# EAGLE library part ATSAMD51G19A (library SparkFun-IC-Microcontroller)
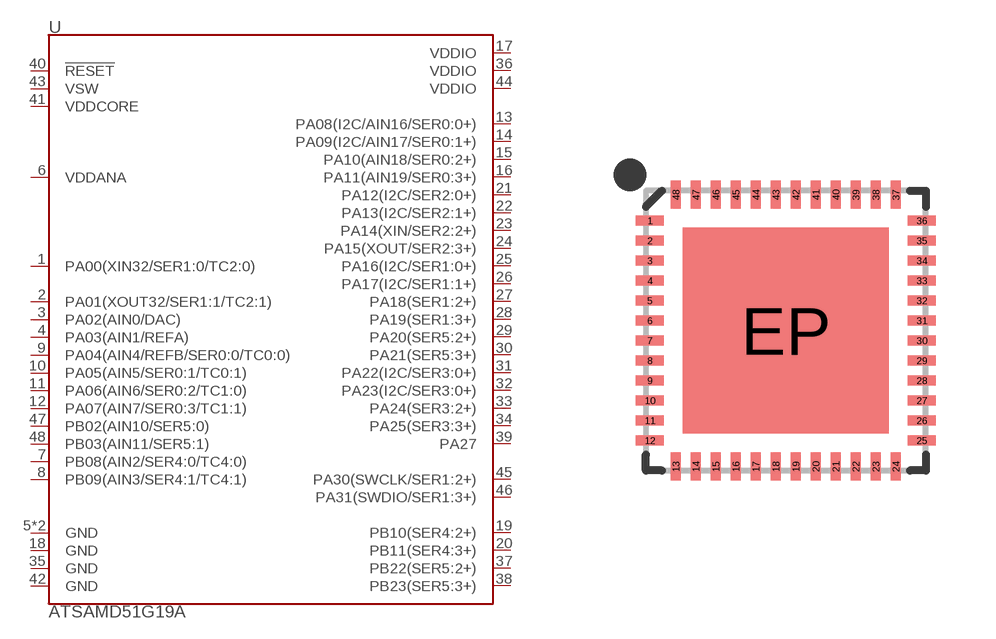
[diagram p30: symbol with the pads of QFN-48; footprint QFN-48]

Designator prefix -

## ATSAMD51G19A  [QFN-48]
1  PA00(XIN32/SER1:0/TC2:0)
2  PA01(XOUT32/SER1:1/TC2:1)
3  PA02(AIN0/DAC)
4  PA03(AIN1/REFA)
5  GND
6  VDDANA
7  PB08(AIN2/SER4:0/TC4:0)
8  PB09(AIN3/SER4:1/TC4:1)
9  PA04(AIN4/REFB/SER0:0/TC0:0)
10  PA05(AIN5/SER0:1/TC0:1)
11  PA06(AIN6/SER0:2/TC1:0)
12  PA07(AIN7/SER0:3/TC1:1)
13  PA08(I2C/AIN16/SER0:0+)
14  PA09(I2C/AIN17/SER0:1+)
15  PA10(AIN18/SER0:2+)
16  PA11(AIN19/SER0:3+)
17  VDDIO
18  GND
19  PB10(SER4:2+)
20  PB11(SER4:3+)
21  PA12(I2C/SER2:0+)
22  PA13(I2C/SER2:1+)
23  PA14(XIN/SER2:2+)
24  PA15(XOUT/SER2:3+)
25  PA16(I2C/SER1:0+)
26  PA17(I2C/SER1:1+)
27  PA18(SER1:2+)
28  PA19(SER1:3+)
29  PA20(SER5:2+)
30  PA21(SER5:3+)
31  PA22(I2C/SER3:0+)
32  PA23(I2C/SER3:0+)
33  PA24(SER3:2+)
34  PA25(SER3:3+)
35  GND
36  VDDIO
37  PB22(SER5:2+)
38  PB23(SER5:3+)
39  PA27
40  !RESET!
41  VDDCORE
42  GND
43  VSW
44  VDDIO
45  PA30(SWCLK/SER1:2+)
46  PA31(SWDIO/SER1:3+)
47  PB02(AIN10/SER5:0)
48  PB03(AIN11/SER5:1)
EP  GND

## Footprint QFN-48 (pad centres in mm)
48-pin QFN (7x7mm, 0.5mm pitch) Used on: ATSAMD21G
smd 0.7 x 0.25: 1 -3.4,2.75; 2 -3.4,2.25; 3 -3.4,1.75; 4 -3.4,1.25; 5 -3.4,0.75; 6 -3.4,0.25; 7 -3.4,-0.25; 8 -3.4,-0.75; 9 -3.4,-1.25; 10 -3.4,-1.75; 11 -3.4,-2.25; 12 -3.4,-2.75; 25 3.4,-2.75; 26 3.4,-2.25; 27 3.4,-1.75; 28 3.4,-1.25; 29 3.4,-0.75; 30 3.4,-0.25; 31 3.4,0.25; 32 3.4,0.75; 33 3.4,1.25; 34 3.4,1.75; 35 3.4,2.25; 36 3.4,2.75
smd 0.25 x 0.7: 13 -2.75,-3.4; 14 -2.25,-3.4; 15 -1.75,-3.4; 16 -1.25,-3.4; 17 -0.75,-3.4; 18 -0.25,-3.4; 19 0.25,-3.4; 20 0.75,-3.4; 21 1.25,-3.4; 22 1.75,-3.4; 23 2.25,-3.4; 24 2.75,-3.4; 37 2.75,3.4; 38 2.25,3.4; 39 1.75,3.4; 40 1.25,3.4; 41 0.75,3.4; 42 0.25,3.4; 43 -0.25,3.4; 44 -0.75,3.4; 45 -1.25,3.4; 46 -1.75,3.4; 47 -2.25,3.4; 48 -2.75,3.4
smd 5.15 x 5.15: EP 0,0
